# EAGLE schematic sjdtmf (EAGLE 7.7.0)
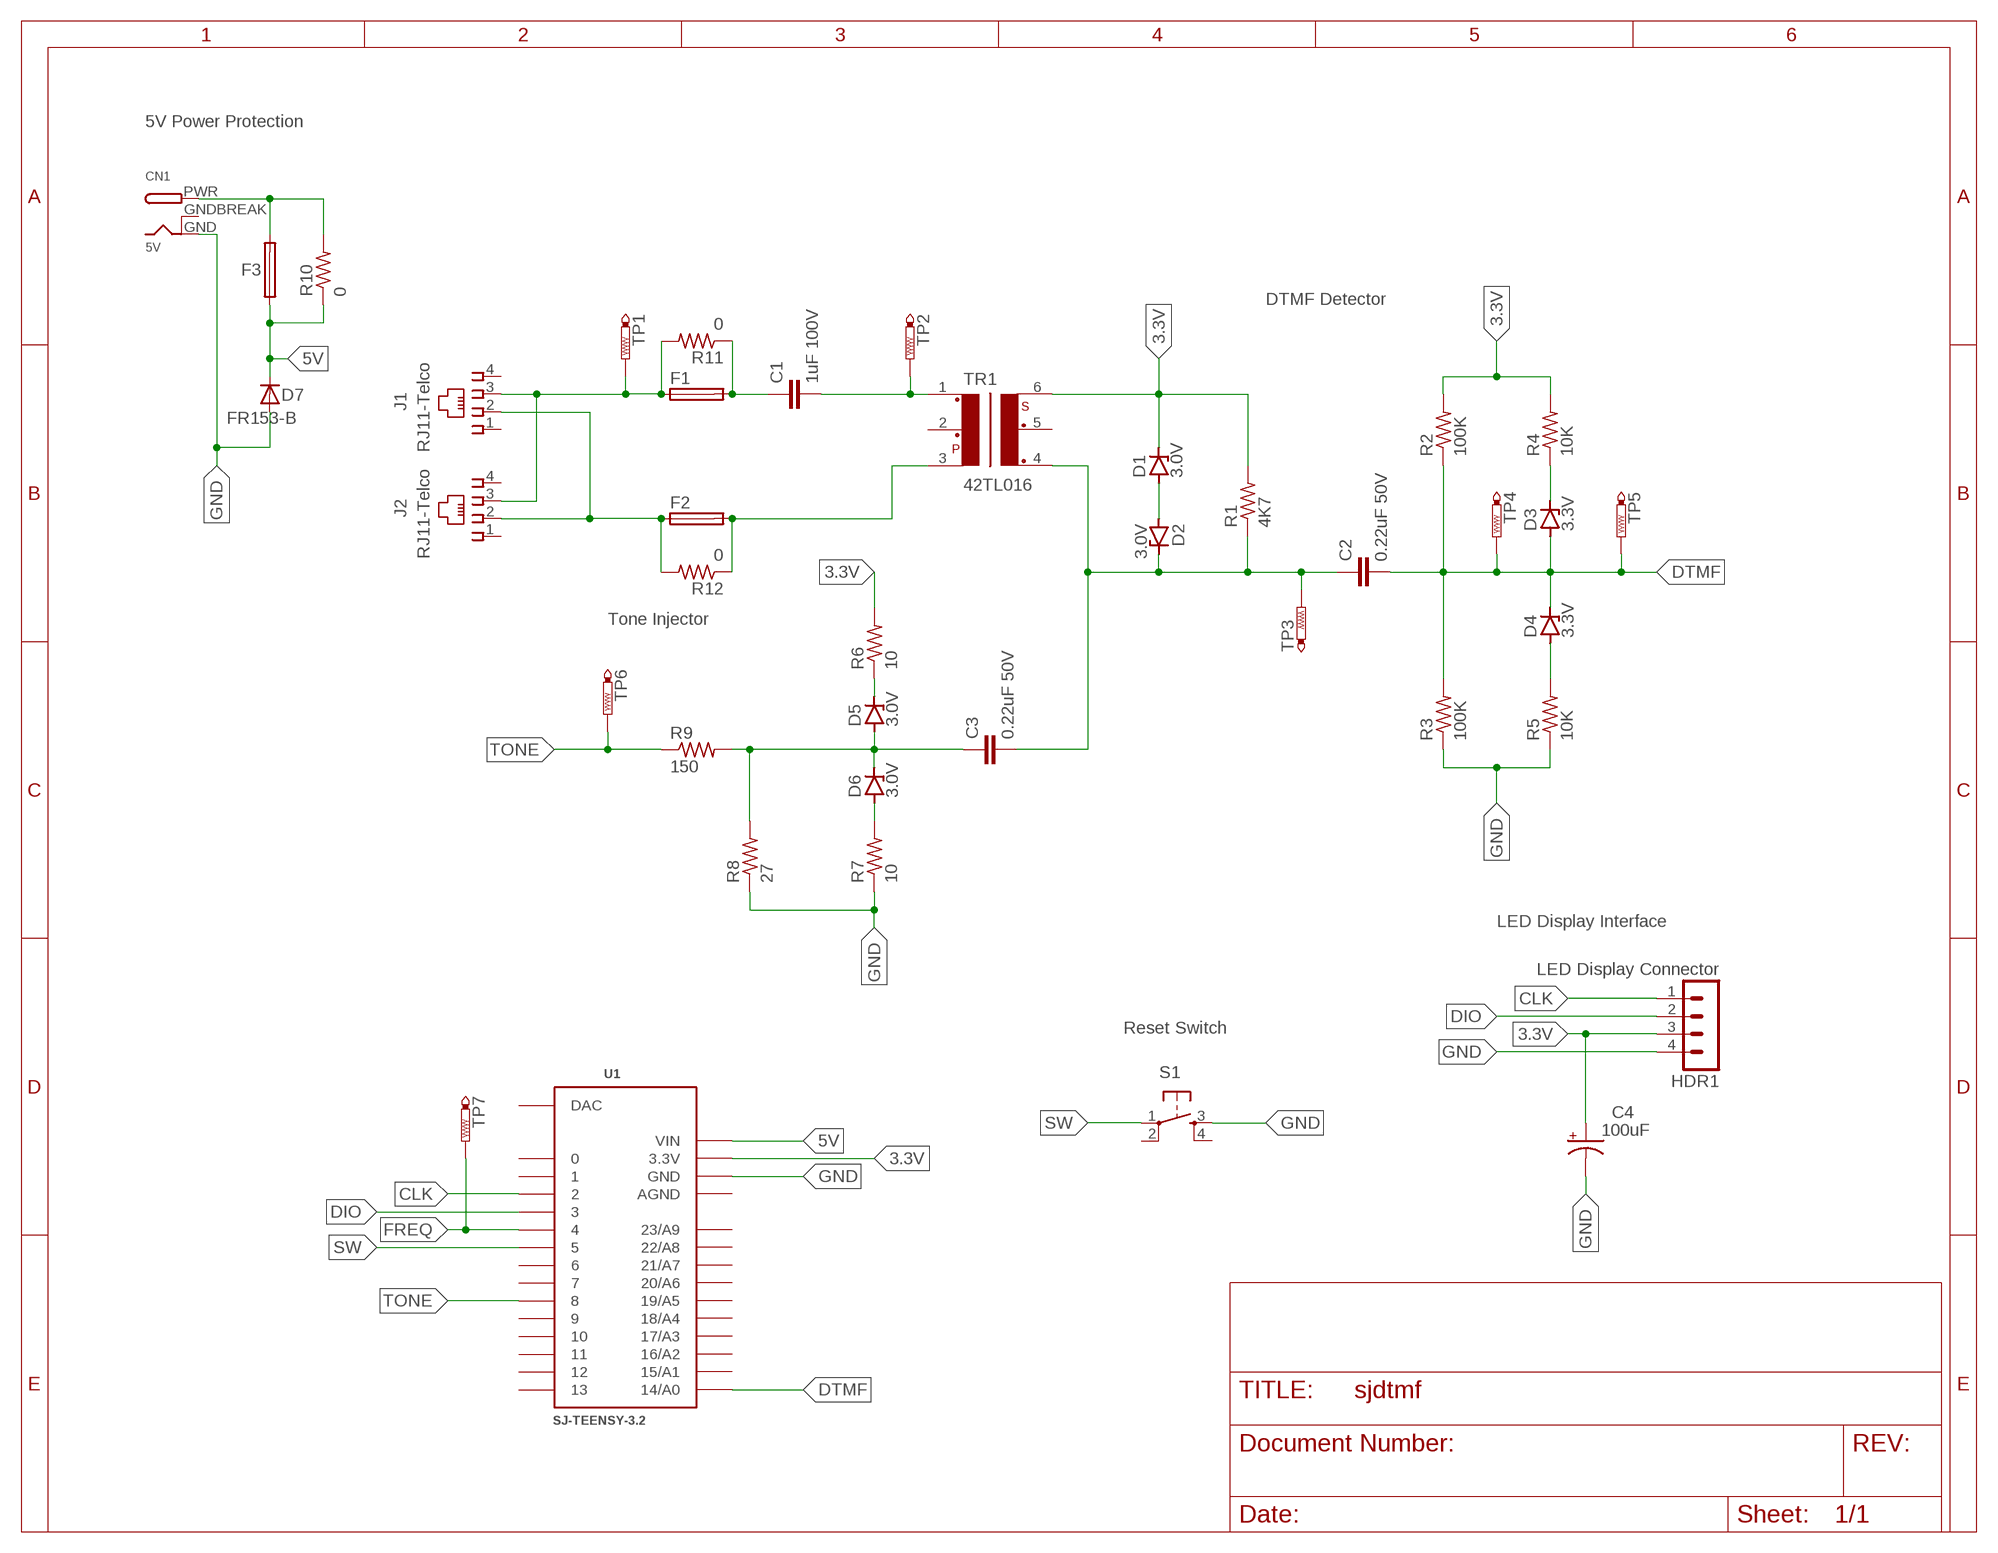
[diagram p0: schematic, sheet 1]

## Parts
C1  1uF 100V  C5/5.5  [C5B5.5]
C2  0.22uF 50V  C5/5.5  [C5B5.5]
C3  0.22uF 50V  C5/5.5  [C5B5.5]
C4  100uF  CPOL-USE2.5-6  [E2,5-6]
CN1  5V  DCBARRELPTH  [DCJACK_2MM_PTH]
D1  3.0V  ZENER-DIODEDO41Z10  [DO41Z10]
D2  3.0V  ZENER-DIODEDO41Z10  [DO41Z10]
D3  3.3V  ZENER-DIODEDO41Z10  [DO41Z10]
D4  3.3V  ZENER-DIODEDO41Z10  [DO41Z10]
D5  3.0V  ZENER-DIODEDO41Z10  [DO41Z10]
D6  3.0V  ZENER-DIODEDO41Z10  [DO41Z10]
D7  FR153-B  DIODE-DO15-12  [DO15-12]
F1  TRF600-150  [TRF600-150]
F2  TRF600-150  [TRF600-150]
F3  6V .75A  RUSBF075  [RUSBF075]
HDR1  LED Display Connector  MA04-1  [MA04-1]
J1  RJ11-Telco  555163-2  [555163-2]
J2  RJ11-Telco  555163-2  [555163-2]
R1  4K7  R-US_0207/10  [0207/10]
R2  100K  R-US_0207/10  [0207/10]
R3  100K  R-US_0207/10  [0207/10]
R4  10K  R-US_0207/10  [0207/10]
R5  10K  R-US_0207/10  [0207/10]
R6  10  R-US_0207/10  [0207/10]
R7  10  R-US_0207/10  [0207/10]
R8  27  R-US_0207/10  [0207/10]
R9  150  R-US_0207/10  [0207/10]
R10  0  R-US_0207/10  [0207/10]
R11  0  R-US_0207/10  [0207/10]
R12  0  R-US_0207/10  [0207/10]
S1  TAC_SWITCHPTH  [TACTILE-PTH]
TP1  PTR1JP-TESTPOINT  [JP-TESTPOINT]
TP2  PTR1JP-TESTPOINT  [JP-TESTPOINT]
TP3  PTR1JP-TESTPOINT  [JP-TESTPOINT]
TP4  PTR1JP-TESTPOINT  [JP-TESTPOINT]
TP5  PTR1JP-TESTPOINT  [JP-TESTPOINT]
TP6  PTR1JP-TESTPOINT  [JP-TESTPOINT]
TP7  PTR1JP-TESTPOINT  [JP-TESTPOINT]
TR1  42TL016  [42TL]
U1  SJ-TEENSY-3.2  [SJ-TEENSY-3.2]

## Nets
3.3V [3V3]: C4.+ D1.C HDR1.3 R1.2 R2.2 R4.2 R6.2 TR1.6 U1.3.3V
5V [5V]: D7.C F3.1 R10.1 U1.VIN
CLK: HDR1.1 U1.2
DIO: HDR1.2 U1.3
DTMF: C2.2 D3.A D4.C R2.1 R3.2 TP4.1(TP) TP5.1(TP) U1.14/A0
FREQ: TP7.1(TP) U1.4
GND: C4.- CN1.GND D7.A HDR1.4 R3.1 R5.1 R7.1 R8.1 S1.3 U1.GND
N$1: C1.1 F1.2 R11.1
N$2 [TelcoSignal]: F1.1 J1.3 J2.3 R11.2 TP1.1(TP)
N$3: C1.2 TP2.1(TP) TR1.1
N$4: F2.2 R12.1 TR1.3
N$5: CN1.PWR F3.2 R10.2
N$6 [TelcoSignal]: F2.1 J1.2 J2.2 R12.2
N$7: D1.A D2.A
N$8: C2.1 C3.2 D2.C R1.1 TP3.1(TP) TR1.4
N$11: D5.C R6.1
N$12: D3.C R4.1
N$13: D4.A R5.2
N$16: C3.1 D5.A D6.C R8.2 R9.2
N$18: D6.A R7.2
SW: S1.1 U1.5
TONE: R9.1 TP6.1(TP) U1.8
Unconnected: J1.1 J1.4 J2.1 J2.4 S1.2 S1.4 TR1.2 TR1.5 U1.0 U1.1 U1.6 U1.7 U1.9 U1.10 U1.11 U1.12 U1.13 U1.15/A1 U1.16/A2 U1.17/A3 U1.18/A4 U1.19/A5 U1.20/A6 U1.21/A7 U1.22/A8 U1.23/A9 U1.DAC

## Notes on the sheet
- 5V Power Protection
- DTMF Detector
- Tone Injector
- LED Display Interface
- Reset Switch

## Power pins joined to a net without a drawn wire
AGND: U1.AGND
GNDBREAK: CN1.GNDBREAK

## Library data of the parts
C1-C3 = capacitor-wima:C: CAPACITOR
C4 = xyfyx:CPOL-US: POLARIZED CAPACITOR, American symbol
CN1 = sj:DCBARREL: 2.0mm DC Barrel Jack DCJACK_2MM_PTH - Through Hole Jack (4UConnector: 05537)
D1-D6 = diode:ZENER-DIODE: Z-Diode
D7 = xyfyx:DIODE-: DIODE
F1 F2 = sj:TRF600-150: TE TRF600-150 .15A 250V DC Fuse
F3 = xyfyx:RUSBF075: RUSBF075 Fuse
HDR1 = con-lstb:MA04-1: PIN HEADER; OC_FARNELL: unknown; OC_NEWARK: unknown
J1 J2 = xyfyx:555163-2: AMP connector
R1-R12 = sj:R-US_: RESISTOR, American symbol
S1 = SparkFun-Retired:TAC_SWITCH: Momentary Switch Button commonly used for reset or general input. Spark Fun Electronics SKU : COM-00097 SMT- SWCH-08247
TP1-TP7 = sj:PTR1: TEST PIN
TR1 = trafo-xicon:42T?*: Xicon Micro-Mini EI-12 Audio Transformers 42TL/42TC/42TM Series Source: http://www.mouser.com//catalog/specsheets/164201.pdf http://www.mouser.com/catalog/specsheets/114225.pdf http://www.mouser.com/catalog/specsheets/164267.pdf; OC_FARNELL: unknown; OC_NEWARK: unknown
U1 = sj:SJ-TEENSY-3.2: SJ Teensy 3.2

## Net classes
1 TelcoSignal: width 0.635 mm, drill 0.305 mm, clearance 2.54 mm
3 5V: width 0.254 mm, drill 0.305 mm, clearance 0.127 mm
4 3V3: width 0.254 mm, drill 0.305 mm, clearance 0.127 mm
